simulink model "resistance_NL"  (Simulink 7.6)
settings: Solver=ode23tb  StartTime=0.0  StopTime=1  RelTol=1e-3
InitFcn:
  | R=100;
StopFcn:
  | close all
  | load I_R_SimPower.mat
  | plot(x(1,:),x(2,:),x(1,:),x(3,:))
  | %axis([0 0.14 -1.2 1.2])
  | grid
  | title('Courant dans R en A et valeur de R en \Omega')
  | xlabel('Simulation d''une résistance dans SimPowerSystems')
libraries: powerlib x7

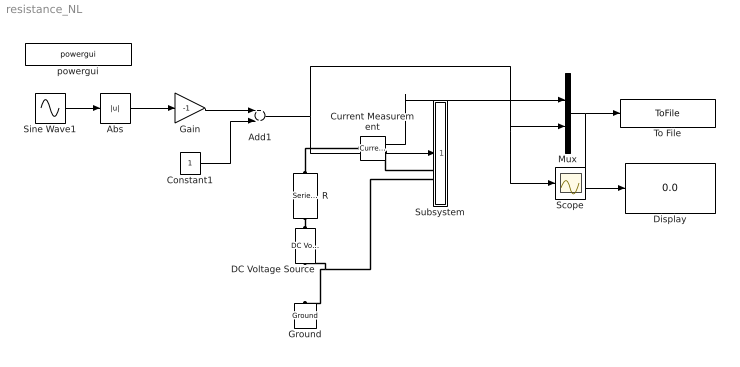
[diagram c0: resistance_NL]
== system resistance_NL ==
  Abs : Abs
  Add1 : Sum  Inputs=+-
  Constant1 : Constant
  Current Measurement : powerlib/Measurements/Current Measurement  DialogController=POWERSYS.PowerSysDialog  SystemSampleTime=-1  PhasorSimulation=off  OutputType=Complex  PSBequivalent=0
  DC Voltage Source : powerlib/Electrical Sources/DC Voltage Source  DialogController=POWERSYS.PowerSysDialog  SystemSampleTime=-1  Amplitude=12  Measurements=None
  Display : Display
  Gain : Gain  Gain=-1
  Ground : powerlib/Elements/Ground  DialogController=POWERSYS.PowerSysDialog  PhysicalDomain=powersysdomain  SubClassName=unknown  LeftPortType=p1  RightPortType=p1  LConnTagsString=a
  Mux : Mux  Inputs=2
  R : powerlib/Elements/Series RLC Branch  DialogController=POWERSYS.PowerSysDialog  PhysicalDomain=powersysdomain  SubClassName=unknown  LeftPortType=p1  RightPortType=p1  LConnTagsString=__new0  RConnTagsString=__new0  BranchType=R  Resistance=0.001  Inductance=10e-3  SetiL0=off  InitialCurrent=0  Capacitance=0  Setx0=off  InitialVoltage=0  Measurements=None
  Scope : Scope
  Sine Wave1 : Sin  Amplitude=5  Frequency=10  SampleTime=0
  Subsystem : Subsystem
  To File : ToFile  Filename=I_R_SimPower  MatrixName=x
  powergui : powerlib/powergui  Priority=1  SystemSampleTime=-1  SimulationMode=Continuous  SampleTime=50e-6  frequency=60  SPID=off  DisableSnubberDevices=off  DisableRonSwitches=off  DisableVfSwitches=off  SwTol=0  Interpol=off  frequencyindice=0  echomessages=off  HookPort=off  DisplayEquations=off  FunctionMessages=off  EnableUseOfTLC=off  x0status=blocks  RestoreLinks=warning  ResistiveCurrentMeasurement=off  Ylog=off  Xlog=on  ShowGrid=off  save=off  variable=ZData  ZoomFFT=off  StartTime=0.0  cycles=1  DisplayStyle=1  fundamental=60  FreqAxis=off  MaxFrequency=1000  frequencyindicesteady=1  display=off  methode=off
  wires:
  Mux/1 -> To File/1, Display/1
  Current Measurement/1 -> Mux/1
  Abs/1 -> Gain/1
  Sine Wave1/1 -> Abs/1
  Constant1/1 -> Add1/2
  Gain/1 -> Add1/1
  Add1/1 -> Subsystem/1(R), Mux/2, Scope/1
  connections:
  Subsystem/LConn2 -- Ground/LConn1 -- DC Voltage Source/LConn1
  Current Measurement/RConn1 -- Subsystem/LConn1
  R/RConn1 -- Current Measurement/LConn1
  DC Voltage Source/RConn1 -- R/LConn1

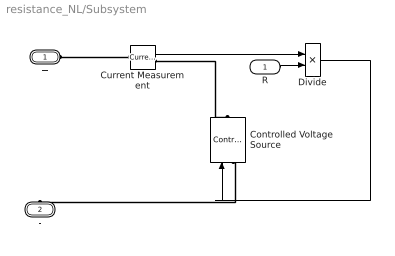
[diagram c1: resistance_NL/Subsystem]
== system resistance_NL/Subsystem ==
  R : Inport
  Controlled Voltage Source : powerlib/Electrical Sources/Controlled Voltage Source  DialogController=POWERSYS.PowerSysDialog  SystemSampleTime=-1  Initialize=on  Source_Type=AC  Amplitude=0  Phase=0  Frequency=0  Measurements=None
  Current Measurement : powerlib/Measurements/Current Measurement  DialogController=POWERSYS.PowerSysDialog  SystemSampleTime=-1  PhasorSimulation=off  OutputType=Complex  PSBequivalent=0
  Divide : Product  Inputs=**
  + : PMIOPort  Port=1  Side=Left
  - : PMIOPort  Port=2  Side=Left
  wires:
  Current Measurement/1 -> Divide/1
  Divide/1 -> Controlled Voltage Source/1
  R/1 -> Divide/2
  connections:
  Current Measurement/RConn1 -- Controlled Voltage Source/RConn1
  +/RConn1 -- Current Measurement/LConn1
  -/RConn1 -- Controlled Voltage Source/LConn1
